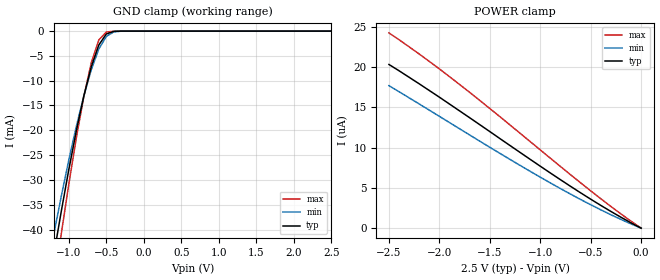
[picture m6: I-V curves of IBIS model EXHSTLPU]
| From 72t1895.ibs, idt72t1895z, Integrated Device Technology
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|   Model EXHSTLPU
[Model]   EXHSTLPU
Model_type   Input
Vinl =  0.400V
Vinh =  1.400V
Vmeas =  0.900V
C_comp   3.00pF   NA   NA
[Temperature Range]   25.00   85.00   -40.00
[Voltage Range]   2.50V   2.30V   2.70V
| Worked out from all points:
|   GND clamp passes 1 mA (typ) near -0.52 V on its own axis
[GND_clamp]
| voltage   I(typ)   I(min)   I(max)
-2.5V     -171mA     -153mA     -195mA
-1.2V     -45.09mA   -40.91mA   -51.21mA
-1.1V     -36.28mA   -33.25mA   -40.8mA
-1V       -27.91mA   -25.98mA   -30.84mA
-900mV    -20.12mA   -19.21mA   -21.55mA
-800mV    -13.11mA   -13.08mA   -13.22mA
-700mV    -7.179mA   -7.775mA   -6.354mA
-600mV    -2.808mA   -3.618mA   -1.788mA
-500mV    -576uA     -1.062mA   -195uA
-400mV    -56.63uA   -160uA     -15.52uA
-300mV    -7.47uA    -16.77uA   -7.499uA
2.5V      50.97pA    1.082uA    -1.591uA
[POWER_clamp]
| voltage   I(typ)   I(min)   I(max)
-2.5V     20.32uA    17.69uA    24.24uA
-2.2V     17.92uA    15.42uA    21.62uA
-1.8V     14.56uA    12.34uA    17.84uA
-900mV    6.85uA     5.617uA    8.684uA
-400mV    2.826uA    2.275uA    3.653uA
0V        50.97pA    2.018nA    220fA
